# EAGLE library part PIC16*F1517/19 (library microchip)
28/40/44-Pin Flash Microcontrollers with nanoWatt XLP Technology PIC16F1517/1519 AND PIC16LF1517/1519 Source: www.microchip.com PIC16F1516.pdf
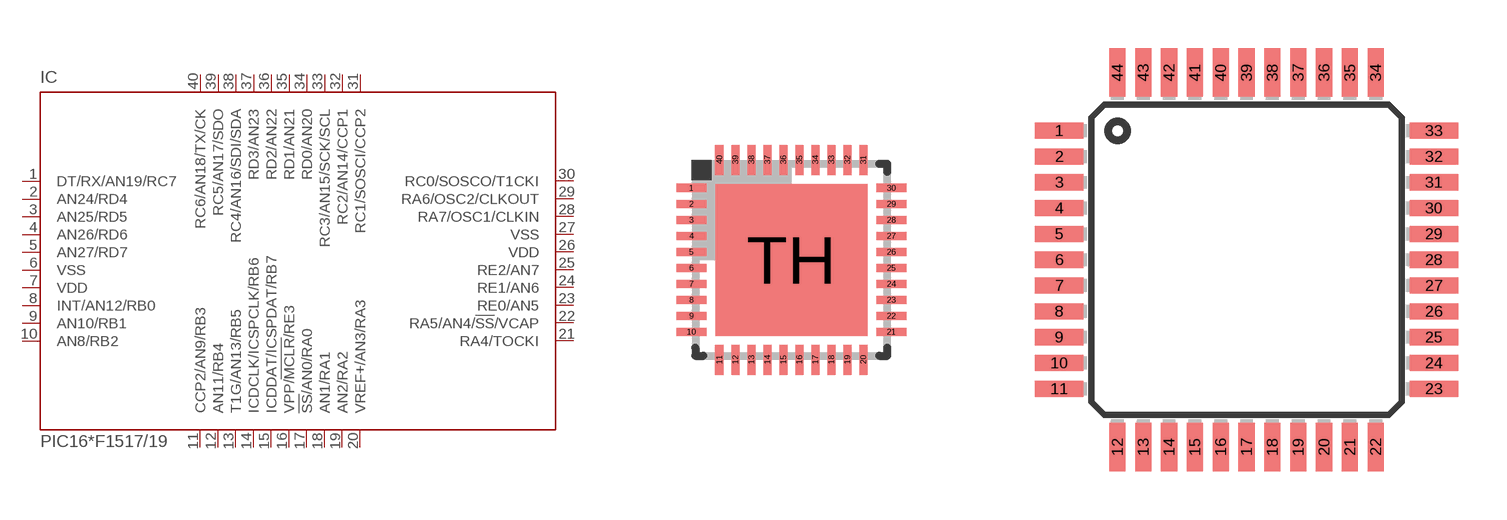
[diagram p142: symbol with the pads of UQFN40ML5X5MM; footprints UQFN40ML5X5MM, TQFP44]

Designator prefix IC

## PIC16F1517/19MV  [UQFN40ML5X5MM]
1  DT/RX/AN19/RC7
2  AN24/RD4
3  AN25/RD5
4  AN26/RD6
5  AN27/RD7
6  VSS  pwr
7  VDD  pwr
8  INT/AN12/RB0
9  AN10/RB1
10  AN8/RB2
11  CCP2/AN9/RB3
12  AN11/RB4
13  T1G/AN13/RB5
14  ICDCLK/ICSPCLK/RB6
15  ICDDAT/ICSPDAT/RB7
16  VPP/!MCLR!/RE3  in
17  !SS!/AN0/RA0
18  AN1/RA1
19  AN2/RA2
20  VREF+/AN3/RA3
21  RA4/TOCKI
22  RA5/AN4/!SS!/VCAP
23  RE0/AN5
24  RE1/AN6
25  RE2/AN7
26  VDD  pwr
27  VSS  pwr
28  RA7/OSC1/CLKIN
29  RA6/OSC2/CLKOUT
30  RC0/SOSCO/T1CKI
31  RC1/SOSCI/CCP2
32  RC2/AN14/CCP1
33  RC3/AN15/SCK/SCL
34  RD0/AN20
35  RD1/AN21
36  RD2/AN22
37  RD3/AN23
38  RC4/AN16/SDI/SDA
39  RC5/AN17/SDO
40  RC6/AN18/TX/CK

## PIC16F1517/19PT  [TQFP44]
1  DT/RX/AN19/RC7
2  AN24/RD4
3  AN25/RD5
4  AN26/RD6
5  AN27/RD7
6  VSS  pwr
7  VDD  pwr
8  INT/AN12/RB0
9  AN10/RB1
10  AN8/RB2
11  CCP2/AN9/RB3
14  AN11/RB4
15  T1G/AN13/RB5
16  ICDCLK/ICSPCLK/RB6
17  ICDDAT/ICSPDAT/RB7
18  VPP/!MCLR!/RE3  in
19  !SS!/AN0/RA0
20  AN1/RA1
21  AN2/RA2
22  VREF+/AN3/RA3
23  RA4/TOCKI
24  RA5/AN4/!SS!/VCAP
25  RE0/AN5
26  RE1/AN6
27  RE2/AN7
28  VDD  pwr
29  VSS  pwr
30  RA7/OSC1/CLKIN
31  RA6/OSC2/CLKOUT
32  RC0/SOSCO/T1CKI
35  RC1/SOSCI/CCP2
36  RC2/AN14/CCP1
37  RC3/AN15/SCK/SCL
38  RD0/AN20
39  RD1/AN21
40  RD2/AN22
41  RD3/AN23
42  RC4/AN16/SDI/SDA
43  RC5/AN17/SDO
44  RC6/AN18/TX/CK

## PIC16F1517/19P, PIC16LF1517/19P  [DIL40]
1  VPP/!MCLR!/RE3  in
2  !SS!/AN0/RA0
3  AN1/RA1
4  AN2/RA2
5  VREF+/AN3/RA3
6  RA4/TOCKI
7  RA5/AN4/!SS!/VCAP
8  RE0/AN5
9  RE1/AN6
10  RE2/AN7
11  VDD  pwr
12  VSS  pwr
13  RA7/OSC1/CLKIN
14  RA6/OSC2/CLKOUT
15  RC0/SOSCO/T1CKI
16  RC1/SOSCI/CCP2
17  RC2/AN14/CCP1
18  RC3/AN15/SCK/SCL
19  RD0/AN20
20  RD1/AN21
21  RD2/AN22
22  RD3/AN23
23  RC4/AN16/SDI/SDA
24  RC5/AN17/SDO
25  RC6/AN18/TX/CK
26  DT/RX/AN19/RC7
27  AN24/RD4
28  AN25/RD5
29  AN26/RD6
30  AN27/RD7
31  VSS  pwr
32  VDD  pwr
33  INT/AN12/RB0
34  AN10/RB1
35  AN8/RB2
36  CCP2/AN9/RB3
37  AN11/RB4
38  T1G/AN13/RB5
39  ICDCLK/ICSPCLK/RB6
40  ICDDAT/ICSPDAT/RB7

## Footprint UQFN40ML5X5MM (pad centres in mm)
40-Lead Platic Ultra Thin Quad Flat, No Lead Package (MV) - 5x5mm Body [UQFN] Source: www.microchip.com PIC16F1516.pdf
smd 0.75 x 0.2: 1 -2.5,1.8; 2 -2.5,1.4; 3 -2.5,1; 4 -2.5,0.6; 5 -2.5,0.2; 6 -2.5,-0.2; 7 -2.5,-0.6; 8 -2.5,-1; 9 -2.5,-1.4; 10 -2.5,-1.8; 21 2.5,-1.8; 22 2.5,-1.4; 23 2.5,-1; 24 2.5,-0.6; 25 2.5,-0.2; 26 2.5,0.2; 27 2.5,0.6; 28 2.5,1; 29 2.5,1.4; 30 2.5,1.8
smd 0.2 x 0.75: 11 -1.8,-2.5; 12 -1.4,-2.5; 13 -1,-2.5; 14 -0.6,-2.5; 15 -0.2,-2.5; 16 0.2,-2.5; 17 0.6,-2.5; 18 1,-2.5; 19 1.4,-2.5; 20 1.8,-2.5; 31 1.8,2.5; 32 1.4,2.5; 33 1,2.5; 34 0.6,2.5; 35 0.2,2.5; 36 -0.2,2.5; 37 -0.6,2.5; 38 -1,2.5; 39 -1.4,2.5; 40 -1.8,2.5
smd 3.8 x 3.8: TH 0,0

## Footprint TQFP44 (pad centres in mm)
Thin Quad Flat Pack package type TQ
smd 1.5 x 0.5: 1 -5.8,4; 2 -5.8,3.2; 3 -5.8,2.4; 4 -5.8,1.6; 5 -5.8,0.8; 6 -5.8,0; 7 -5.8,-0.8; 8 -5.8,-1.6; 9 -5.8,-2.4; 10 -5.8,-3.2; 11 -5.8,-4; 23 5.8,-4; 24 5.8,-3.2; 25 5.8,-2.4; 26 5.8,-1.6; 27 5.8,-0.8; 28 5.8,0; 29 5.8,0.8; 30 5.8,1.6; 31 5.8,2.4; 32 5.8,3.2; 33 5.8,4
smd 0.5 x 1.5: 12 -4,-5.8; 13 -3.2,-5.8; 14 -2.4,-5.8; 15 -1.6,-5.8; 16 -0.8,-5.8; 17 0,-5.8; 18 0.8,-5.8; 19 1.6,-5.8; 20 2.4,-5.8; 21 3.2,-5.8; 22 4,-5.8; 34 4,5.8; 35 3.2,5.8; 36 2.4,5.8; 37 1.6,5.8; 38 0.8,5.8; 39 0,5.8; 40 -0.8,5.8; 41 -1.6,5.8; 42 -2.4,5.8; 43 -3.2,5.8; 44 -4,5.8

## Footprint DIL40 (pad centres in mm)
Dual In Line package type P
drill 0.813 long: 1 -24.13,-7.62; 2 -21.59,-7.62; 3 -19.05,-7.62; 4 -16.51,-7.62; 5 -13.97,-7.62; 6 -11.43,-7.62; 7 -8.89,-7.62; 8 -6.35,-7.62; 9 -3.81,-7.62; 10 -1.27,-7.62; 11 1.27,-7.62; 12 3.81,-7.62; 13 6.35,-7.62; 14 8.89,-7.62; 15 11.43,-7.62; 16 13.97,-7.62; 17 16.51,-7.62; 18 19.05,-7.62; 19 21.59,-7.62; 20 24.13,-7.62; 21 24.13,7.62; 22 21.59,7.62; 23 19.05,7.62; 24 16.51,7.62; 25 13.97,7.62; 26 11.43,7.62; 27 8.89,7.62; 28 6.35,7.62; 29 3.81,7.62; 30 1.27,7.62; 31 -1.27,7.62; 32 -3.81,7.62; 33 -6.35,7.62; 34 -8.89,7.62; 35 -11.43,7.62; 36 -13.97,7.62; 37 -16.51,7.62; 38 -19.05,7.62; 39 -21.59,7.62; 40 -24.13,7.62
